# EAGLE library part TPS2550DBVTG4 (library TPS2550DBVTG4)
USB Power SW Hi Side/DIST Single 6.5V 0.1A to 1.1A 6-Pin SOT-23 T/R Source: Datasheet
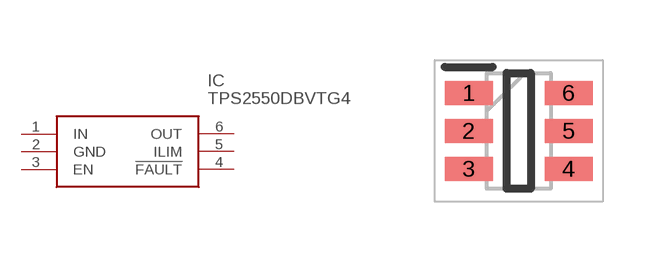
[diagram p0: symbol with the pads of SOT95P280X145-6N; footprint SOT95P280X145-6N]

Designator prefix IC

## TPS2550DBVTG4 (Arrow_Part_Number: TPS2550DBVTG4; Arrow_Price-Stock: https://www.arrow.com/en/products/tps2550dbvtg4/texas-instruments; Description: USB Power SW Hi Side/DIST Single 6.5V 0.1A to 1.1A 6-Pin SOT-23 T/R; Height: 1.45mm; Manufacturer_Name: Texas Instruments; Manufacturer_Part_Number: TPS2550DBVTG4; Mouser_Part_Number: 595-TPS2550DBVTG4; Mouser_Price-Stock: https://www.mouser.co.uk/ProductDetail/Texas-Instruments/TPS2550DBVTG4?qs=ql1K%252BkDau3qOVhP421dR5A%3D%3D)  [SOT95P280X145-6N]
1  IN
2  GND
3  EN
4  !FAULT
5  ILIM
6  OUT

## Footprint SOT95P280X145-6N (pad centres in mm)
DBV0006A
smd 1.2 x 0.6: 1 -1.25,0.95; 2 -1.25,0; 3 -1.25,-0.95; 4 1.25,-0.95; 5 1.25,0; 6 1.25,0.95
